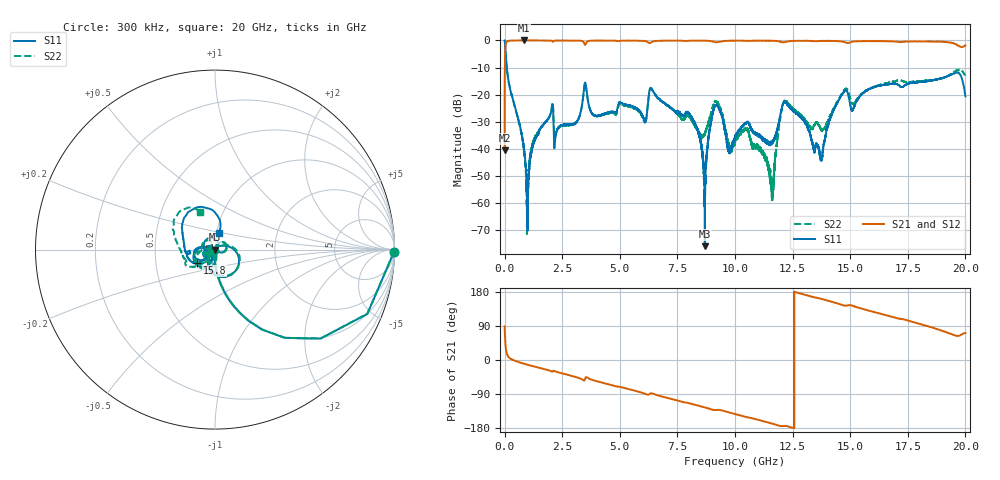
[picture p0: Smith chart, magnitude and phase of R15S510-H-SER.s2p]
!{R15S510}
!Johanson Technology Inc.
!www.johansontechnology.com
!Test Board Conditions:
!Substrate Type  RO4350B
!Substrate Thickness  20 mil
!Substrate Dk  3.66
!TL Type: GCPW
!TL Trace Width  34 mil
!TL Gap  10 mil
!Electrode orientation  Horizontal
!DUT TOPOLOGY	SERIES
!Mounting Pad LxW  26x52 mil
! Created Sat Feb  6 14:31:46 2021
# hz S ma R 50
! 2 Port Network Data from SP1.SP block
! freq  magS11  angS11  magS21  angS21  magS12  angS12  magS22  angS22
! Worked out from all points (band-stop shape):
!   20001 points, 300 kHz to 20 GHz, reference 50 ohm
!   highest |S21| = 0.00 dB at 837.3 MHz (marker M1); lowest = -40.5 dB at 300 kHz (marker M2)
!   |S21| within 3 dB of the highest: 31.86 MHz to end of sweep
!   lowest |S11| = -75.9 dB at 8.691 GHz (marker M3), VSWR 1.00, Z = 50 - j0.0154 ohm
!   |S11| at or under -10 dB: 94.18 MHz to end of sweep
!   |S22| runs from -71.4 to 0.0 dB; largest |S21 - S12| = 0.013
!   S11 on the Smith chart (normalised r, x): 300 kHz: open; 15.8 GHz: 0.81, -0.12; 20 GHz: 1.02, +0.19
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300000  0.9977 -0.7  0.00947 88.8  0.009506 89.6  0.9975 -0.6
1.203e8  0.2519 -77.0  0.9668 13.0  0.9668 13.0  0.2526 -76.7
8.373e8  0.01025 -101.9  0.9998 -9.8  0.9983 -9.9  0.009587 -101.4
1.0053e9  0.001046 111.1  0.999 -12.7  0.9992 -12.7  0.002085 94.3
1.2663e9  0.01306 76.8  0.9989 -16.9  0.9991 -16.9  0.01428 75.1
2.0103e9  0.04643 56.6  0.993 -29.1  0.9929 -29.1  0.04679 54.0
2.2313e9  0.01922 58.6  0.9958 -30.8  0.9955 -30.8  0.01944 44.7
3.3343e9  0.05571 22.7  0.9836 -50.2  0.9831 -50.2  0.0552 26.9
6.6673e9  0.08708 175.1  0.9845 -93.5  0.985 -93.5  0.08472 -172.0
8.0613e9  0.04071 151.1  0.9876 -114.9  0.989 -114.9  0.03647 -179.4
8.6913e9  0.0001605 -74.0  0.989 -125.2  0.9883 -125.1  0.01901 -104.1
9.1563e9  0.0633 -120.8  0.9294 -131.9  0.9312 -131.9  0.07517 -106.7
1.00003e10  0.01695 -98.8  0.9897 -142.6  0.99 -142.6  0.01372 -61.2
1.05073e10  0.03004 -109.9  0.9835 -150.8  0.9847 -150.7  0.0223 -52.0
1.16003e10  0.01359 -149.1  0.9861 -167.7  0.9859 -167.6  0.00145 -48.6
1.21433e10  0.0729 138.2  0.9262 -173.8  0.9264 -173.9  0.0759 164.9
1.33343e10  0.01401 47.9  0.9811 167.2  0.9803 167.1  0.02323 153.3
1.37423e10  0.006288 -16.6  0.9784 161.5  0.9807 161.5  0.02225 179.6
1.46903e10  0.1068 -148.9  0.9494 144.4  0.9465 144.6  0.1127 -136.5
1.57983e10  0.126 -143.5  0.9704 130.5  0.9754 130.5  0.1255 -135.0
1.66673e10  0.1552 -161.8  0.9683 116.2  0.9588 116.1  0.1662 -144.8
2e10  0.09307 77.6  0.8123 71.0  0.8091 70.9  0.2248 111.9
